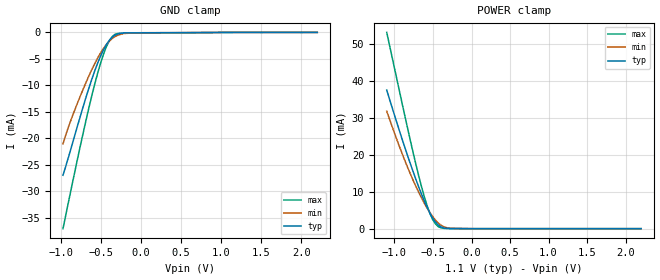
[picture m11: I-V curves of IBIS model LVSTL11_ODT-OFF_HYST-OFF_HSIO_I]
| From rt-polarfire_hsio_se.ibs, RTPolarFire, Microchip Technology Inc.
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|   Model LVSTL11_ODT-OFF_HYST-OFF_HSIO_I
[Model]   LVSTL11_ODT-OFF_HYST-OFF_HSIO_I
Model_type   Input
Vinl =   0.083
Vinh =   0.283
|   typ   min   max
C_comp_pullup   1.335e-12   1.335e-12   1.380e-12
C_comp_pulldown  1.335e-12   1.335e-12   1.380e-12
[Temperature Range]  25C   125C   -55C
[Voltage Range]  1.1   1.045   1.155
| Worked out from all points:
|   GND clamp passes 1 mA (typ) near -0.37 V on its own axis
|   POWER clamp passes 1 mA (typ) near -0.43 V on its own axis
[GND Clamp]
| Voltage   I(typ)   I(min)   I(max)
-974.5mV  -27mA      -21.08mA   -37.09mA
-902.3mV  -23.38mA   -17.69mA   -31.79mA
-794.1mV  -17.7mA    -13.36mA   -23.97mA
-685.8mV  -12.19mA   -9.403mA   -16.51mA
-577.5mV  -7.235mA   -5.867mA   -9.722mA
-505.3mV  -4.465mA   -3.878mA   -5.816mA
-433.1mV  -2.307mA   -2.287mA   -2.708mA
-397mV    -1.509mA   -1.664mA   -1.576mA
-324.8mV  -519.5uA   -776.3uA   -368.5uA
-216.6mV  -119.1uA   -201.6uA   -113.6uA
-36.09mV  -76.1uA    -65.22uA   -96.34uA
2.2V      0A         0A         0A
[POWER Clamp]
| Voltage   I(typ)   I(min)   I(max)
-1.1V     37.55mA    31.83mA    53.19mA
-974.5mV  29.1mA     24.45mA    41.08mA
-866.2mV  22.09mA    18.54mA    30.7mA
-758mV    15.47mA    13.14mA    20.64mA
-649.7mV  9.39mA     8.369mA    11.44mA
-577.5mV  5.839mA    5.618mA    6.29mA
-541.4mV  4.291mA    4.396mA    4.192mA
-505.3mV  2.944mA    3.295mA    2.516mA
-433.1mV  1.016mA    1.546mA    573.6uA
-360.9mV  204.5uA    522.8uA    81.54uA
-252.7mV  30.1uA     83.69uA    30.28uA
2.2V      0A         0A         0A
